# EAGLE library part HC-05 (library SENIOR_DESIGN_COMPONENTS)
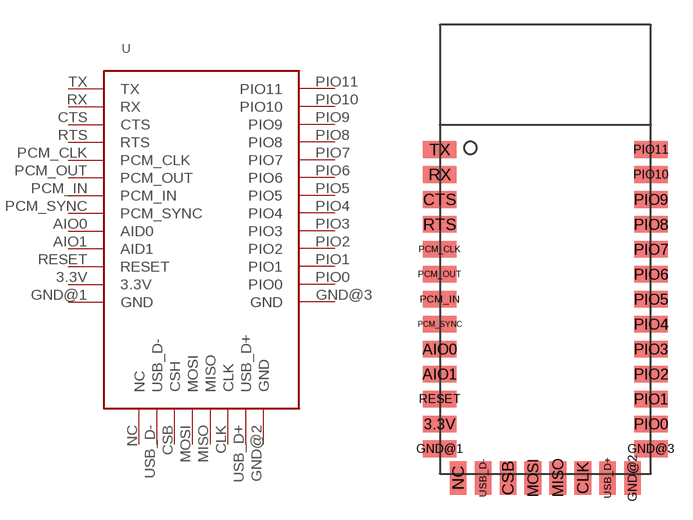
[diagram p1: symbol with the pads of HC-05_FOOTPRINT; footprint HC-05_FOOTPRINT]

Designator prefix -

## HC-05  [HC-05_FOOTPRINT]
3.3V  3.3V
AIO0  AID0
AIO1  AID1
CLK  CLK
CSB  CSH
CTS  CTS
GND@1  GND
GND@2  GND
GND@3  GND
MISO  MISO
MOSI  MOSI
NC  NC
PCM_CLK  PCM_CLK
PCM_IN  PCM_IN
PCM_OUT  PCM_OUT
PCM_SYNC  PCM_SYNC
PIO0  PIO0
PIO1  PIO1
PIO2  PIO2
PIO3  PIO3
PIO4  PIO4
PIO5  PIO5
PIO6  PIO6
PIO7  PIO7
PIO8  PIO8
PIO9  PIO9
PIO10  PIO10
PIO11  PIO11
RESET  RESET
RTS  RTS
RX  RX
TX  TX
USB_D+  USB_D+
USB_D-  USB_D-

## Footprint HC-05_FOOTPRINT (pad centres in mm)
HC-05 Footprint
smd 2 x 1: 3.3V 0,3; AIO0 0,7.5; AIO1 0,6; CTS 0,16.5; GND@1 0,1.5; GND@3 12.7,1.5; PCM_CLK 0,13.5; PCM_IN 0,10.5; PCM_OUT 0,12; PCM_SYNC 0,9; PIO0 12.7,3; PIO1 12.7,4.5; PIO2 12.7,6; PIO3 12.7,7.5; PIO4 12.7,9; PIO5 12.7,10.5; PIO6 12.7,12; PIO7 12.7,13.5; PIO8 12.7,15; PIO9 12.7,16.5; PIO10 12.7,18; PIO11 12.7,19.5; RESET 0,4.5; RTS 0,15; RX 0,18; TX 0,19.5
smd 1 x 2: CLK 8.6,-0.25; CSB 4.1,-0.25; GND@2 11.6,-0.25; MISO 7.1,-0.25; MOSI 5.6,-0.25; NC 1.1,-0.25; USB_D+ 10.1,-0.25; USB_D- 2.6,-0.25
